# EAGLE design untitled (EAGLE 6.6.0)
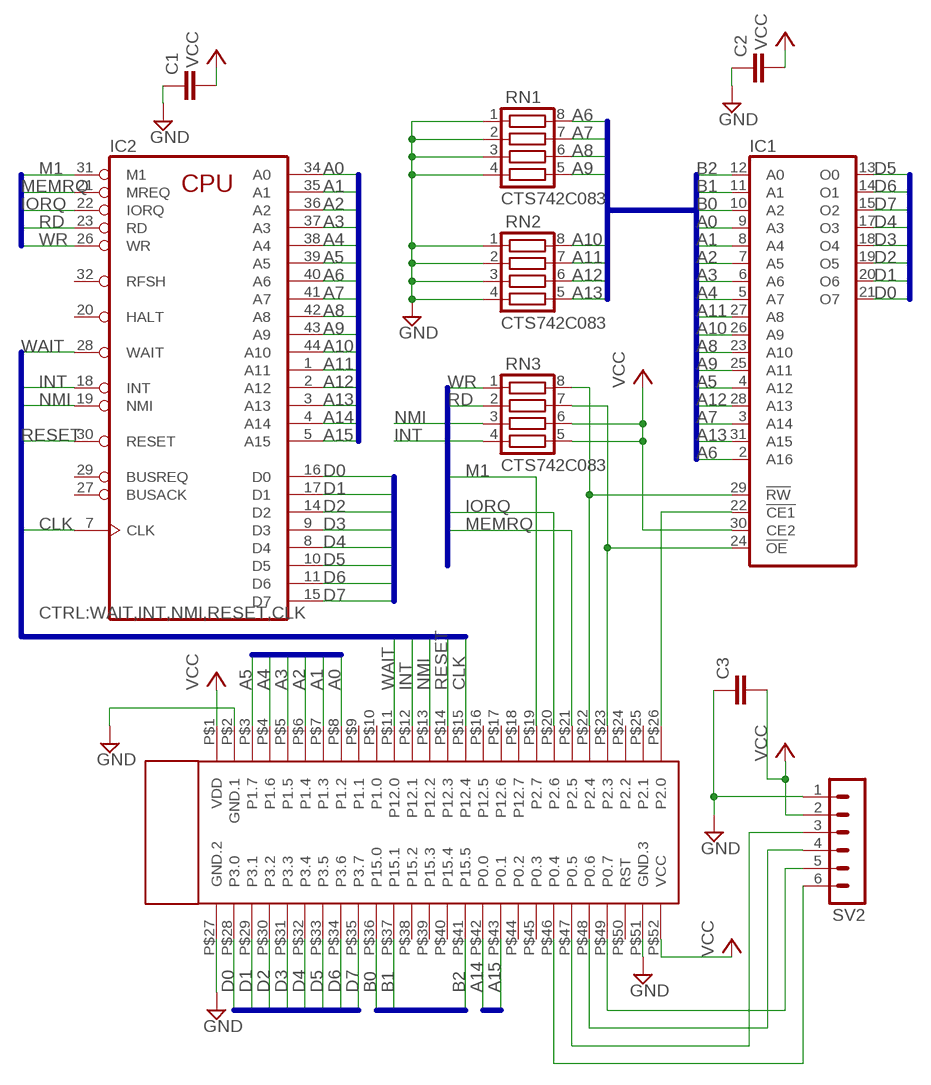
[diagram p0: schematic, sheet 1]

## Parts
C1  C-EUC0805  [C0805]
C2  C-EUC0805  [C0805]
C3  C-EUC0805  [C0805]
IC1  TC551001CF  [SOP32L]
IC2  Z80CPU-FPLCC  [PLCC-44]
RN1  CTS742C083  [CTS742C083]
RN2  CTS742C083  [CTS742C083]
RN3  CTS742C083  [CTS742C083]
SV2  MA06-1  [MA06-1]
U$1  CY8CKIT-059  [CY8CKIT-059]

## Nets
A0: IC1.9(A3) IC2.34(A0) U$1.P$8(P1.2)
A1: IC1.8(A4) IC2.35(A1) U$1.P$7(P1.3)
A2: IC1.7(A5) IC2.36(A2) U$1.P$6(P1.4)
A3: IC1.6(A6) IC2.37(A3) U$1.P$5(P1.5)
A4: IC1.5(A7) IC2.38(A4) U$1.P$4(P1.6)
A5: IC1.4(A12) IC2.39(A5) U$1.P$3(P1.7)
A6: IC1.2(A16) IC2.40(A6) RN1.8
A7: IC1.3(A14) IC2.41(A7) RN1.7
A8: IC1.23(A10) IC2.42(A8) RN1.6
A9: IC1.25(A11) IC2.43(A9) RN1.5
A10: IC1.26(A9) IC2.44(A10) RN2.8
A11: IC1.27(A8) IC2.1(A11) RN2.7
A12: IC1.28(A13) IC2.2(A12) RN2.6
A13: IC1.31(A15) IC2.3(A13) RN2.5
A14: IC2.4(A14) U$1.P$42(P0.0)
A15: IC2.5(A15) U$1.P$43(P0.1)
B0: IC1.10(A2) U$1.P$36(P15.0)
B1: IC1.11(A1) U$1.P$37(P15.1)
B2: IC1.12(A0) U$1.P$41(P15.5)
CLK: IC2.7(CLK) U$1.P$15(P12.4)
D0: IC1.21(O7) IC2.16(D0) U$1.P$28(P3.0)
D1: IC1.20(O6) IC2.17(D1) U$1.P$29(P3.1)
D2: IC1.19(O5) IC2.14(D2) U$1.P$30(P3.2)
D3: IC1.18(O4) IC2.9(D3) U$1.P$31(P3.3)
D4: IC1.17(O3) IC2.8(D4) U$1.P$32(P3.4)
D5: IC1.13(O0) IC2.10(D5) U$1.P$33(P3.5)
D6: IC1.14(O1) IC2.11(D6) U$1.P$34(P3.6)
D7: IC1.15(O2) IC2.15(D7) U$1.P$35(P3.7)
GND: C1.1 C2.1 C3.1 RN1.1 RN1.2 RN1.3 RN1.4 RN2.1 RN2.2 RN2.3 RN2.4 SV2.1 U$1.P$2(GND.1) U$1.P$27(GND.2) U$1.P$51(GND.3)
INT: IC2.18(INT) RN3.4 U$1.P$12(P12.1)
IORQ: IC2.22(IORQ) U$1.P$20(P2.6)
M1: IC2.31(M1) U$1.P$19(P2.7)
MEMRQ: IC2.21(MREQ) U$1.P$21(P2.5)
N$3: SV2.3 U$1.P$47(P0.5)
N$4: SV2.4 U$1.P$48(P0.6)
N$5: SV2.5 U$1.P$49(P0.7)
N$6: SV2.6 U$1.P$46(P0.4)
N$8: IC1.24(!OE) RN3.7 U$1.P$23(P2.3)
N$11: IC1.29(!RW) RN3.8 U$1.P$22(P2.4)
N$13: IC1.22(!CE1) U$1.P$26(P2.0)
NMI: IC2.19(NMI) RN3.3 U$1.P$13(P12.2)
RD: IC2.23(RD) RN3.2
RESET: IC2.30(RESET) U$1.P$14(P12.3)
VCC: C1.2 C2.2 C3.2 IC1.30(CE2) RN3.5 RN3.6 SV2.2 U$1.P$1(VDD) U$1.P$52(VCC)
WAIT: IC2.28(WAIT) U$1.P$11(P12.0)
WR: IC2.26(WR) RN3.1
Unconnected: IC1.1(NC) IC2.6(NC) IC2.12(NC) IC2.20(HALT) IC2.24(NC) IC2.25(NC) IC2.27(BUSACK) IC2.29(BUSREQ) IC2.32(RFSH) U$1.P$9(P1.1) U$1.P$10(P1.0) U$1.P$16(P12.5) U$1.P$17(P12.6) U$1.P$18(P12.7) U$1.P$24(P2.2) U$1.P$25(P2.1) U$1.P$38(P15.2) U$1.P$39(P15.3) U$1.P$40(P15.4) U$1.P$44(P0.2) U$1.P$45(P0.3) U$1.P$50(RST)

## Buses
A[0..15],B[0..2]
D[0..7]
CTRL:WAIT,INT,NMI,RESET,CLK
BUSCTRL:M1,IORQ,MEMRQ,RD,WR
B[0..2]

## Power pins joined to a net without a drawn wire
GND: IC1.16(GND) IC2.33(GND)
VCC: IC1.32(VCC) IC2.13(VCC)

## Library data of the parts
C1-C3 = resistor:C-EU: CAPACITOR, European symbol
IC1 = memory:TC551001CF: MEMORY
IC2 = Z80FAMIL:Z80CPU-F
RN1-RN3 = resistor-net:CTS742C083: Chip Resistor Array 4 Single Resistor Source: http://www.ctscorp.com/components/Datasheets/CTSChipArrayDs.pdf; OC_FARNELL: unknown; OC_NEWARK: unknown
SV2 = con-lstb:MA06-1: PIN HEADER; OC_FARNELL: unknown; OC_NEWARK: unknown
U$1 = untitled:CY8CKIT-059

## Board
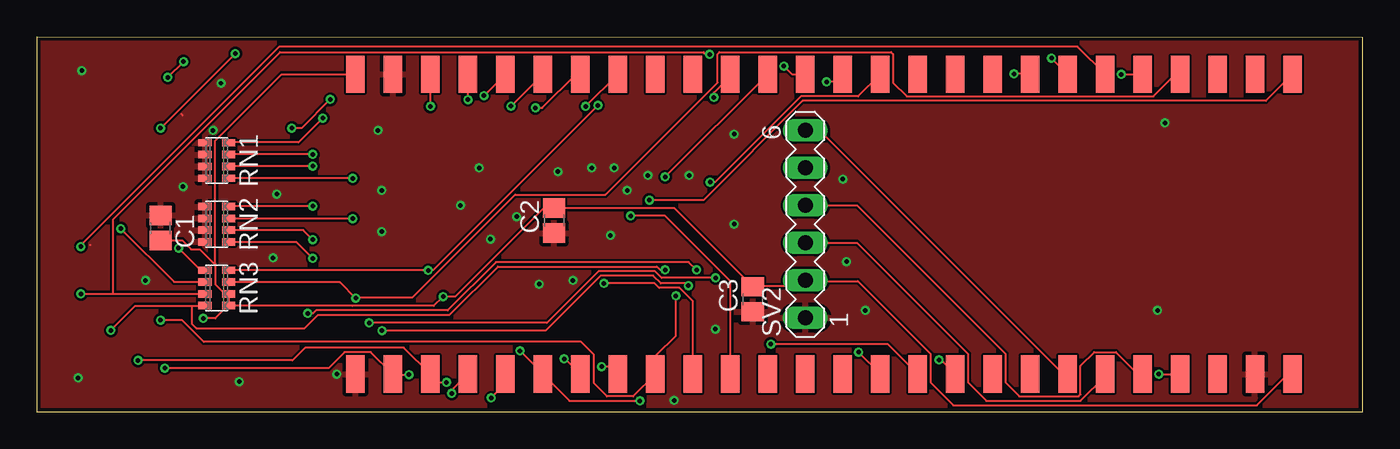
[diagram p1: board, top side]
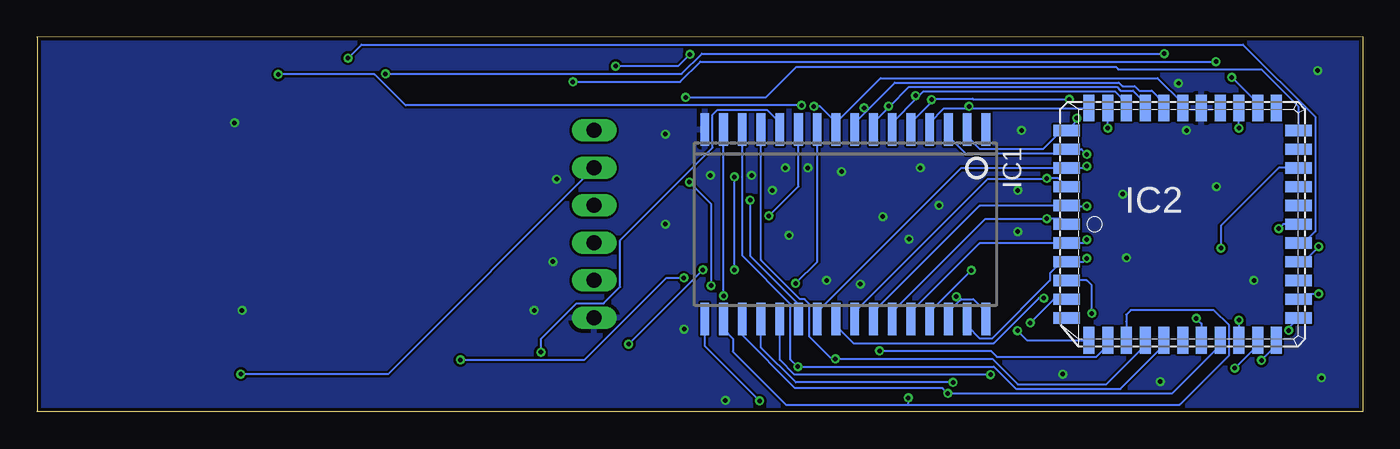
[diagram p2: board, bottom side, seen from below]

Size 89.84 x 25.39 mm. Coordinates in mm from the lower left corner, seen from the top.
Outline: 89.84,0 0,0 0,25.39 89.84,25.38
Outline: 89.81,25.36 89.81,0.03
Copper layers (1*16): Top 0.035mm / dielectric 1.5mm / Bottom 0.035mm
Design rules "SeeedStudio_2layer_DRU_no_angle_20140221": minimum track width 6mil, minimum drill 12mil, track to track 6mil, track to pad 6mil, pad to pad 6mil, via to via 6mil, smd to smd 0mil, copper to edge 10mil, drill to drill 10mil, minimum pad ring 10mil, minimum via ring 6mil, stop-mask expansion 2mil, vias tented up to drill 100mil, thermal gap 10mil

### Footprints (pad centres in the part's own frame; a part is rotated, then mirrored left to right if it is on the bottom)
C0805 = smd 1.3 x 1.5: 1 -0.85,0; 2 0.85,0
SOP32L = smd 0.6 x 2.2: 1 -9.525,-6.416; 2 -8.255,-6.416; 3 -6.985,-6.416; 4 -5.715,-6.416; 5 -4.445,-6.416; 6 -3.175,-6.416; 7 -1.905,-6.416; 8 -0.635,-6.416; 9 0.635,-6.416; 10 1.905,-6.416; 11 3.175,-6.416; 12 4.445,-6.416; 13 5.715,-6.416; 14 6.985,-6.416; 15 8.255,-6.416; 16 9.525,-6.416; 17 9.525,6.416; 18 8.255,6.416; 19 6.985,6.416; 20 5.715,6.416; 21 4.445,6.416; 22 3.175,6.416; 23 1.905,6.416; 24 0.635,6.416; 25 -0.635,6.416; 26 -1.905,6.416; 27 -3.175,6.416; 28 -4.445,6.416; 29 -5.715,6.416; 30 -6.985,6.416; 31 -8.255,6.416; 32 -9.525,6.416
PLCC-44 = smd 1.8 x 0.76: 1 -7.86,0; 2 -7.86,-1.27; 3 -7.86,-2.54; 4 -7.86,-3.81; 5 -7.86,-5.08; 6 -7.86,-6.35; 18 7.86,-6.35; 19 7.86,-5.08; 20 7.86,-3.81; 21 7.86,-2.54; 22 7.86,-1.27; 23 7.86,0; 24 7.86,1.27; 25 7.86,2.54; 26 7.86,3.81; 27 7.86,5.08; 28 7.86,6.35; 40 -7.86,6.35; 41 -7.86,5.08; 42 -7.86,3.81; 43 -7.86,2.54; 44 -7.86,1.27 | smd 0.76 x 1.8: 7 -6.35,-7.86; 8 -5.08,-7.86; 9 -3.81,-7.86; 10 -2.54,-7.86; 11 -1.27,-7.86; 12 0,-7.86; 13 1.27,-7.86; 14 2.54,-7.86; 15 3.81,-7.86; 16 5.08,-7.86; 17 6.35,-7.86; 29 6.35,7.86; 30 5.08,7.86; 31 3.81,7.86; 32 2.54,7.86; 33 1.27,7.86; 34 0,7.86; 35 -1.27,7.86; 36 -2.54,7.86; 37 -3.81,7.86; 38 -5.08,7.86; 39 -6.35,7.86
CTS742C083 = smd 0.5 x 0.9: 1 -1.2,-0.8; 2 -0.4,-0.8; 3 0.4,-0.8; 4 1.2,-0.8; 5 1.2,0.8; 6 0.4,0.8; 7 -0.4,0.8; 8 -1.2,0.8
MA06-1 = drill 1.016 long: 1 -6.35,0; 2 -3.81,0; 3 -1.27,0; 4 1.27,0; 5 3.81,0; 6 6.35,0
CY8CKIT-059 = smd 1.27 x 2.54: P$1 -33.02,10.16; P$2 -30.48,10.16; P$3 -27.94,10.16; P$4 -25.4,10.16; P$5 -22.86,10.16; P$6 -20.32,10.16; P$7 -17.78,10.16; P$8 -15.24,10.16; P$9 -12.7,10.16; P$10 -10.16,10.16; P$11 -7.62,10.16; P$12 -5.08,10.16; P$13 -2.54,10.16; P$14 0,10.16; P$15 2.54,10.16; P$16 5.08,10.16; P$17 7.62,10.16; P$18 10.16,10.16; P$19 12.7,10.16; P$20 15.24,10.16; P$21 17.78,10.16; P$22 20.32,10.16; P$23 22.86,10.16; P$24 25.4,10.16; P$25 27.94,10.16; P$26 30.48,10.16; P$27 -33.02,-10.16; P$28 -30.48,-10.16; P$29 -27.94,-10.16; P$30 -25.4,-10.16; P$31 -22.86,-10.16; P$32 -20.32,-10.16; P$33 -17.78,-10.16; P$34 -15.24,-10.16; P$35 -12.7,-10.16; P$36 -10.16,-10.16; P$37 -7.62,-10.16; P$38 -5.08,-10.16; P$39 -2.54,-10.16; P$40 0,-10.16; P$41 2.54,-10.16; P$42 5.08,-10.16; P$43 7.62,-10.16; P$44 10.16,-10.16; P$45 12.7,-10.16; P$46 15.24,-10.16; P$47 17.78,-10.16; P$48 20.32,-10.16; P$49 22.86,-10.16; P$50 25.4,-10.16; P$51 27.94,-10.16; P$52 30.48,-10.16

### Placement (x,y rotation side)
C1  8.38,12.45 270 top
C2  35.05,12.95 90 top
C3  48.51,7.62 90 top
IC1  35.05,12.7 180 bottom
IC2  12.19,12.7 0 bottom
RN1  12.19,17.02 270 top
RN2  12.19,12.7 270 top
RN3  12.19,8.38 270 top
SV2  52.07,12.7 90 top
U$1  54.61,12.7 0 top

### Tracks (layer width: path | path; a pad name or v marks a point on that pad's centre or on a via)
A0  (via drill 0.3)
  Top 0.152: v37.19,20.68 U$1.P$8
  Bottom 0.152: IC2.34 12.19,20.9 13.89,22.61 32.66,22.61 35.69,19.58 IC1.9 35.74,19.63 36.78,20.68 v37.19,20.68
A1  (via drill 0.3)
  Top 0.152: U$1.P$7 36.52,22.86 34.24,20.57 v33.78,20.57
  Bottom 0.152: IC2.35 13.46,20.9 14.3,21.74 15.14,21.74 15.44,22.05 16.28,22.05 16.54,22.3 31.7,22.3 33.6,20.4 | 33.6,20.4 34.42,19.58 IC1.8 | 33.6,20.4 v33.78,20.57
A2  (via drill 0.3)
  Top 0.152: v32.13,20.7 U$1.P$6
  Bottom 0.152: IC2.36 14.73,20.9 15.57,21.74 16.41,21.74 16.66,22 30.73,22 32.08,20.65 | 32.08,20.65 33.15,19.58 IC1.7 | v32.13,20.7 32.08,20.65
A3  (via drill 0.3)
  Top 0.152: v30.3,21.41 U$1.P$5
  Bottom 0.152: IC2.37 16,20.9 16.79,21.69 29.77,21.69 30.18,21.29 | 30.18,21.29 31.88,19.58 IC1.6 | 30.18,21.29 v30.3,21.41
A4  (via drill 0.3)
  Top 0.152: v17.27,19.2 17.93,19.2 v19.89,21.16 | v29.21,21.13 U$1.P$4
  Bottom 0.152: v17.27,19.2 IC2.38 | v19.89,21.16 26.39,21.16 26.44,21.21 28.98,21.21 29.13,21.06 | 29.13,21.06 30.61,19.58 IC1.5 | v29.21,21.13 29.13,21.06
A5  (via drill 0.3)
  Top 0.152: v26.67,20.68 U$1.P$3
  Bottom 0.152: 26.67,20.55 28.37,20.55 29.34,19.58 IC1.4 | 26.67,20.55 18.54,20.55 IC2.39 | 26.67,20.55 v26.67,20.68
A6  (via drill 0.3)
  Top 0.152: v19.38,19.89 17.73,18.24 13.01,18.24 RN1.8
  Bottom 0.152: v19.38,19.89 19.38,19.71 IC2.40 20.12,19.02 20.42,19.02 21.67,17.78 25.93,17.78 26.8,18.64 IC1.2
A7  (via drill 0.3)
  Top 0.152: v18.69,17.42 13.01,17.42 RN1.7
  Bottom 0.152: v18.69,17.42 19.05,17.78 IC2.41 20.12,17.75 20.4,17.48 26.9,17.48 28.07,18.64 IC1.3
A8  (via drill 0.3)
  Top 0.152: v18.69,16.64 13.01,16.64 RN1.6
  Bottom 0.152: v18.69,16.64 18.82,16.51 IC2.42 20.12,16.48 27.23,16.48 36.96,6.76 IC1.23
A9  (via drill 0.3)
  Top 0.152: v21.41,15.8 13.01,15.8 RN1.5
  Bottom 0.152: IC2.43 20.07,15.24 20.62,15.8 v21.41,15.8 21.46,15.75 25.43,15.75 34.42,6.76 IC1.25
A10  (via drill 0.3)
  Top 0.152: v18.69,13.92 13.01,13.92 RN2.8
  Bottom 0.152: v18.69,13.92 19.99,13.92 IC2.44 20.12,13.95 25.96,13.95 33.15,6.76 IC1.26
A11  (via drill 0.3)
  Top 0.152: v21.41,13.08 13.01,13.08 RN2.7
  Bottom 0.152: IC2.1 20.07,12.7 20.45,13.08 v21.41,13.08 21.46,13.03 25.6,13.03 31.88,6.76 IC1.27
A12  (via drill 0.3)
  Top 0.152: v18.69,11.66 18.06,12.29 13.01,12.29 RN2.6
  Bottom 0.152: v18.69,11.66 18.92,11.43 IC2.2 20.12,11.4 25.96,11.4 30.61,6.76 IC1.28
A13  (via drill 0.3)
  Top 0.152: v18.69,10.39 17.6,11.48 13.01,11.48 RN2.5
  Bottom 0.152: v18.69,10.39 18.92,10.16 IC2.3 20.12,10.13 20.42,10.13 21.18,9.37 21.18,8.89 25.12,4.95 25.93,4.95 26.8,5.82 IC1.31
A14  (via drill 0.3)
  Top 0.152: v18.36,6.66 18.72,6.66 18.92,6.86 27.84,6.86 31.11,10.13 44.17,10.13 v44.7,9.6 | v49.73,4.57 57.66,4.57 U$1.P$42
  Bottom 0.152: IC2.4 18.69,8.89 18.36,8.56 v18.36,6.66 | v49.73,4.57 v44.7,9.6
A15  (via drill 0.3)
  Top 0.152: v22.53,6.02 34.57,6.02 38.08,9.53 41.88,9.53 42.34,9.07 v46,9.07 | v61.14,3.5 61.27,3.5 U$1.P$43
  Bottom 0.152: IC2.5 20.93,7.62 v22.53,6.02 | v46,9.07 47.17,9.07 52.73,3.5 v61.14,3.5
B0  (via drill 0.3)
  Top 0.152: v38.43,8.69 41.86,8.69 42.16,8.38 43.54,8.38 44.45,7.47 U$1.P$36
  Bottom 0.152: IC1.10 36.96,10.16 v38.43,8.69
B1  (via drill 0.3)
  Top 0.152: v40.23,13.26 42.57,13.26 46.99,8.84 U$1.P$37
  Bottom 0.152: IC1.11 38.23,15.27 v40.23,13.26
B2  (via drill 0.3)
  Top 0.152: v55.68,4.04 57.15,2.56 U$1.P$41
  Bottom 0.152: IC1.12 39.5,19.58 40.36,20.45 43.71,20.45 44.04,20.12 44.04,17.88 50.32,11.61 50.32,8.46 51.44,7.34 53.26,7.34 55.68,4.93 v55.68,4.04
CLK  (via drill 0.3)
  Top 0.152: v23.39,5.49 34.47,5.49 38.2,9.22 41.76,9.22 42.29,8.69 43.99,8.69 v44.15,8.53 | v45.62,15.54 45.95,15.54 51.77,21.36 55.65,21.36 U$1.P$15
  Bottom 0.152: v23.39,5.49 22.76,4.85 IC2.7 | v44.15,8.53 44.15,14.07 v45.62,15.54
D0  (via drill 0.3)
  Top 0.152: v8.66,2.95 19.76,2.95 20.85,4.04 22.63,4.04 U$1.P$28 24.18,2.52 v25.22,2.52
  Bottom 0.152: IC2.16 7.11,4.5 v8.66,2.95 | IC1.21 39.5,3.5 38.51,2.52 v25.22,2.52
D1  (via drill 0.3)
  Top 0.152: v6.86,3.48 17.32,3.48 18.19,4.34 24.87,4.34 U$1.P$29 27.23,1.98 v27.76,1.98
  Bottom 0.152: IC2.17 5.84,4.5 v6.86,3.48 | IC1.20 40.77,4.34 38.41,1.98 v27.76,1.98
D2  (via drill 0.3)
  Top 0.152: v28.12,1.25 28.12,1.45 U$1.P$30
  Bottom 0.152: IC2.14 9.65,4.5 12.9,1.25 v28.12,1.25 28.47,1.6 38.46,1.6 42.04,5.18 IC1.19
D3  (via drill 0.3)
  Top 0.152: U$1.P$31 31.75,1.91 v30.79,0.94
  Bottom 0.152: 43.31,5.59 IC1.18 43.26,5.54 42.67,4.95 42.67,4.06 39.09,0.48 30.79,0.48 | IC2.9 16,6.1 16.03,6.12 16.03,6.58 15.72,6.88 10.08,6.88 9.04,5.84 9.04,3.83 12.39,0.48 30.79,0.48 | 30.79,0.48 v30.79,0.94
D4  (via drill 0.3)
  Top 0.152: v32.74,4.12 34.29,2.56 U$1.P$32 36.09,0.74 v40.87,0.74
  Bottom 0.152: IC2.8 17.27,4.5 18.06,3.71 24.79,3.71 25.2,4.12 v32.74,4.12 | IC1.17 44.58,4.45 v40.87,0.74
D5  (via drill 0.3)
  Top 0.152: v35.74,3.58 35.79,3.58 U$1.P$33
  Bottom 0.152: IC2.10 14.73,4.5 17.37,1.85 23.37,1.85 25.09,3.58 v35.74,3.58 35.79,3.63 36.04,3.63 37.49,5.08 37.49,7.29 37.82,7.62 38.12,7.62 40.77,10.26 IC1.13
D6  (via drill 0.3)
  Top 0.152: v38.28,3.05 38.86,3.05 U$1.P$34
  Bottom 0.152: IC2.11 13.46,4.5 16.41,1.55 23.5,1.55 24.99,3.05 v38.28,3.05 38.76,3.53 38.76,7.29 42.04,10.57 IC1.14
D7  (via drill 0.3)
  Top 0.152: v8.38,6.2 9.83,6.2 11.3,4.72 36.88,4.72 37.74,3.86 37.74,1.93 38.63,1.04 40.41,1.04 U$1.P$35 41.96,2.59 41.96,3.81 43.31,5.16 v43.31,7.85
  Bottom 0.152: v8.38,6.2 IC2.15 | v43.31,7.85 IC1.15
GND  (via drill 0.3)
  Top 0.152: 3.61,11.3 3.63,11.3 | 9.78,20.17 9.87,20.08
  Bottom 0.152: IC2.33 10.77,21.06 10.92,21.06
  other vias: 2.79,2.29 3.05,23.11 7.37,8.89 16,10.41 47.24,12.7 35.31,16.26 47.24,18.8 36.32,8.89 38.86,11.94 37.59,16.51 23.11,19.05 13.72,2.03 11.94,19.05 29.97,16.51 41.4,16 39.12,16.51 75.95,6.86 76.45,19.56 54.61,15.75 54.86,10.16 56.13,6.86 28.7,13.97 23.37,12.19 23.37,14.99 34.04,8.64 45.97,5.59 43.18,0.76 16.26,14.73 9.91,15.24 20.32,2.54 32.51,13.21 30.73,11.68 44.2,16 40.01,14.99 12.47,22.25
  pour Top: 0,25.4 90.17,25.4 90.17,0 0,0
  pour Bottom: 0,0 0,25.4 89.92,25.4 89.92,0
INT  (via drill 0.3)
  Top 0.152: 10.49,7.16 6.66,7.16 v5,5.51 | 10.49,7.16 11.38,7.16 RN3.4 | v42.57,15.9 U$1.P$12 | v42.57,9.6 42.24,9.6 42.01,9.83 31.24,9.83 27.96,6.55 19.05,6.55 18.16,5.66 10.79,5.66 10.49,5.97 10.49,7.16
  Bottom 0.152: v5,5.51 5,5.69 4.34,6.35 IC2.18 | v42.57,9.6 v42.57,15.9
IORQ  (via drill 0.3)
  Top 0.152: U$1.P$20 v68.76,23.95
  Bottom 0.152: IC2.22 3.99,11.43 3.2,12.22 3.2,19.96 8.1,24.87 67.84,24.87 v68.76,23.95
M1  (via drill 0.3)
  Top 0.152: v13.44,24.26 v8.38,19.2 | v66.22,22.89 67.28,22.89 U$1.P$19
  Bottom 0.152: v8.38,19.2 IC2.31 | v13.44,24.26 44.78,24.26 46.15,22.89 v66.22,22.89
MEMRQ  (via drill 0.3)
  Top 0.152: v2.97,11.18 2.97,11.28 16.43,24.74 70.51,24.74 U$1.P$21
  Bottom 0.152: IC2.21 3.99,10.16 v2.97,11.18
N$3
  Top 0.152: U$1.P$47 72.39,2.41 70.71,0.74 64.34,0.74 63.09,1.98 63.09,3.91 55.58,11.43 SV2.3
N$4
  Top 0.152: U$1.P$48 74.62,2.54 73.13,4.04 71.65,4.04 70.71,3.1 70.71,1.17 70.59,1.04 66.57,1.04 65.63,1.98 65.63,3.91 55.58,13.97 SV2.4
N$5  (via drill 0.3)
  Top 0.152: v76.02,2.54 U$1.P$49
  Bottom 0.152: v76.02,2.54 66.04,2.54 SV2.5
N$6
  Top 0.152: U$1.P$46 69.55,2.54 53.03,19.05 SV2.6
N$8  (via drill 0.3)
  Top 0.152: RN3.7 13.01,8.76 20.55,8.76 v21.61,7.7 21.67,7.75 25.45,7.75 32.41,14.71 38.53,14.71 46.13,22.3 46.13,24.23 46.25,24.36 57.89,24.36 58.01,24.23 58.01,22.3 58.95,21.36 75.67,21.36 77.17,22.86 U$1.P$23
  Bottom 0.152: v21.61,7.7 21.95,7.7 24.99,4.65 34.52,4.65 35.69,5.82 IC1.24
N$11  (via drill 0.3)
  Top 0.152: RN3.8 13.01,9.58 v26.52,9.58 26.57,9.63 26.9,9.63 v38.02,20.75 | v73.48,22.86 U$1.P$22
  Bottom 0.152: v26.52,9.58 29.34,6.76 IC1.29 | v73.48,22.86 66.95,22.86 64.85,20.75 v38.02,20.75
N$13  (via drill 0.3)
  Top 0.152: v41.5,14.33 45.16,14.33 51.89,21.06 83.29,21.06 U$1.P$26
  Bottom 0.152: IC1.22 38.23,7.29 41.5,10.57 v41.5,14.33
NMI  (via drill 0.3)
  Top 0.152: v2.97,7.98 5.16,7.98 | 5.16,7.98 11.38,7.98 RN3.3 | U$1.P$13 51.18,22.86 v50.62,23.42 | v45.59,24.21 45.34,24.21 45.19,24.36 16.48,24.36 5.16,13.03 5.16,7.98
  Bottom 0.152: v2.97,7.98 3.96,7.98 4.32,7.62 IC2.19 | v50.62,23.42 46.38,23.42 v45.59,24.21
RD  (via drill 0.3)
  Top 0.152: v5.69,12.39 9.3,8.79 11.38,8.79 RN3.2
  Bottom 0.152: v5.69,12.39 5.38,12.7 IC2.23
RESET  (via drill 0.3)
  Top 0.152: v9.93,23.72 v8.87,22.66 | v53.52,22.35 54.1,22.35 U$1.P$14
  Bottom 0.152: IC2.30 7.11,20.9 v8.87,22.66 | v9.93,23.72 44.88,23.72 46.25,22.35 v53.52,22.35
VCC  (via drill 0.3)
  Top 0.152: RN3.5 13.01,7.19 13.01,7.98 RN3.6 12.93,8 12.72,8 12.09,8.64 12.09,9.93 12.04,9.98 | 12.04,9.98 11.02,11 10.44,11 9.83,11.61 C1.2 | v11.28,6.33 12.09,6.33 12.93,7.16 RN3.5 | U$1.P$1 16.59,22.86 12.09,18.36 12.09,10.03 12.04,9.98 | U$1.P$52 84.78,2.54 82.68,0.43 62.1,0.43 60.55,1.98 60.55,3.91 55.63,8.84 52.12,8.84 SV2.2 51.66,8.48 48.51,8.48 C3.2 48.46,8.53 43.2,13.79 C2.2 35,13.74 34.29,13.74 28.35,7.8 v27.53,7.8 26.9,7.16 21.39,7.16 21.36,7.19 13.08,7.19 RN3.5
  Bottom 0.152: IC2.13 10.92,5.97 v11.28,6.33 | IC1.32 25.53,6.76 26.39,7.62 27.2,7.62 27.28,7.54 | 27.28,7.54 28.07,6.76 IC1.30 | v27.53,7.8 27.28,7.54
WAIT  (via drill 0.3)
  Top 0.152: v45.87,21.29 45.87,21.61 46.99,22.73 U$1.P$11
  Bottom 0.152: v45.87,21.29 40.44,21.29 38.35,23.37 16.74,23.37 16.56,23.19 6.86,23.19 4.34,20.68 4.34,19.05 IC2.28
WR  (via drill 0.3)
  Top 0.152: v9.6,11.07 11.07,9.6 11.38,9.6 RN3.1
  Bottom 0.152: v9.6,11.07 9.6,12.6 5.69,16.51 IC2.26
